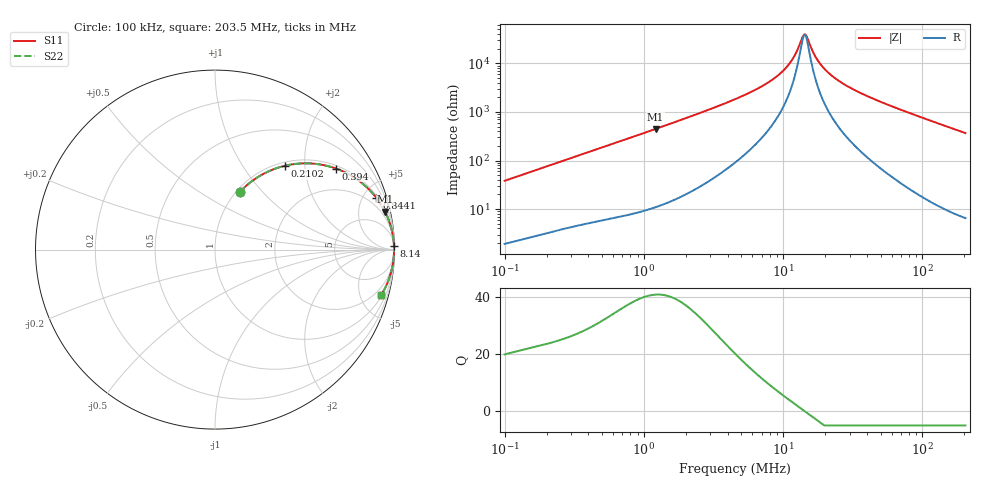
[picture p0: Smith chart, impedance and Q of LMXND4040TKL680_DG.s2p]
! LMXND4040TKL680_DG  S-PARAMETER MODEL  ( General Type )
! Model Generated by TAIYO YUDEN Corporation (https://www.yuden.co.jp/en/)
! Version 1.0
! TAIYO YUDEN Control No. 191023NI43SB-FBB
! Copyright(c) 2019 TAIYO YUDEN CO.,LTD. All Rights Reserved.
! Product Description (link to TY-COMPAS)
! https://ds.yuden.co.jp/TYCOMPAS/or/detail?pn=LMXND4040TKL680MDG&u=M
! Products Name : Inductors
! Characteristics :
!  Inductance : 68 uH , SRF(min) : 8.3 MHz , DC Resistance(max) : 1.2 Ohm
!  Rated Current : Saturation :520 mA , Temp Rise : 320 mA (40 degC)
!  Case Size : 4.0 x 4.0 / 0.157 x 0.157 [mm/inch] , Thickness : 1.8 / 0.071 [mm/inch]
!  (Conditions: Temperature = 25 degC , DC Bias Current/Voltage = 0A / 0V)
! External Node Assignments :
!  1  o---GGG---o  2
! GND o---------o GND
! Frequency Range : 0.1MHz  -  203.457813MHz  [ 402 STEP ]
# MHz S RI R 50
! Freq[MHz].  S11 Real  S11 Imag  S21 Real  S21 Imag  S12 Real  S12 Imag  S22 Real  S22 Imag
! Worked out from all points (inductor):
!   401 points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, 100 kHz to 203.5 MHz, reference 50 ohm
!   read as one part in series: L = 60.4 uH near 103.9 kHz
!   highest Q = 40.8 at 1.212 MHz (marker M1), where L = 58.5 uH
!   self-resonance near 14.14 MHz
!   S11 on the Smith chart (normalised r, x): 100 kHz: 1.04, +0.76; 210.2 kHz: 1.07, +1.58; 394 kHz: 1.10, +2.92; 844.1 kHz: 1.16, +6.19; 8.14 MHz: 11, +87; 203.5 MHz: 1.13, -7.34
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0.1  0.1394 0.3221  0.8606 -0.3221  0.8606 -0.3221  0.1394 0.3221
0.210173  0.3884 0.4668  0.6116 -0.4668  0.6116 -0.4668  0.3884 0.4668
0.358236  0.6337 0.4641  0.3663 -0.4641  0.3663 -0.4641  0.6337 0.4641
0.394026  0.6746 0.4515  0.3254 -0.4515  0.3254 -0.4515  0.6746 0.4515
0.576699  0.8111 0.3767  0.1889 -0.3767  0.1889 -0.3767  0.8111 0.3767
0.844059  0.8996 0.2878  0.1004 -0.2878  0.1004 -0.2878  0.8996 0.2878
1.212063  0.9473 0.2114  0.0527 -0.2114  0.0527 -0.2114  0.9473 0.2114
1.283332  0.9525 0.2007  0.0475 -0.2007  0.0475 -0.2007  0.9525 0.2007
4.51063  0.9943 0.0544  0.00568 -0.0544  0.00568 -0.0544  0.9943 0.0544
8.140366  0.9969 0.0227  0.00307 -0.0227  0.00307 -0.0227  0.9969 0.0227
9.662391  0.9972 0.0153  0.00278 -0.0153  0.00278 -0.0153  0.9972 0.0153
11.04035  0.9974 0.00996  0.00263 -0.00996  0.00263 -0.00996  0.9974 0.00996
12.14336  0.9974 0.00624  0.00257 -0.00624  0.00257 -0.00624  0.9974 0.00624
13.61338  0.9975 0.00184  0.00253 -0.00184  0.00253 -0.00184  0.9975 0.00184
14.14192  0.9975 0.000383  0.00252 -0.000383  0.00252 -0.000383  0.9975 0.000383
14.69098  0.9975 -0.00108  0.00252 0.00108  0.00252 0.00108  0.9975 -0.00108
16.15871  0.9975 -0.00473  0.00254 0.00473  0.00254 0.00473  0.9975 -0.00473
18.81812  0.9974 -0.0107  0.00263 0.0107  0.00263 0.0107  0.9974 -0.0107
24.10469  0.997 -0.0209  0.00297 0.0209  0.00297 0.0209  0.997 -0.0209
33.96119  0.996 -0.0374  0.00396 0.0374  0.00396 0.0374  0.996 -0.0374
57.88634  0.992 -0.0724  0.00796 0.0724  0.00796 0.0724  0.992 -0.0724
203.4578  0.927 -0.2514  0.073 0.2514  0.073 0.2514  0.927 -0.2514
